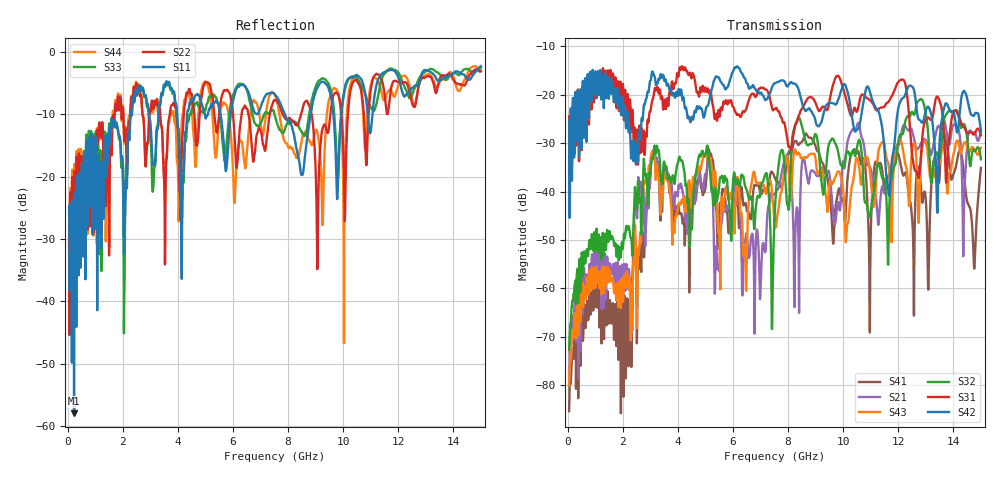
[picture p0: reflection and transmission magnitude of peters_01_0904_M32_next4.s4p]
# MHZ S RI R 50.00
! FREQ  S11  S12  S13  S14
!  S21  S22  S23  S24
!  S31  S32  S33  S34
!  S41  S42  S43  S44
!  REAL  IMAG  REAL  IMAG  REAL  IMAG  REAL  IMAG
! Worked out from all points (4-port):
!   1496 points, 50 MHz to 15 GHz, reference 50 ohm
!   strongest paths, dB at 50 MHz, 3.79 GHz, 7.53 GHz, 11.27 GHz, 15 GHz:
!     S42: -25.4, -20.0, -17.6, -23.3, -27.6
!     S31: -24.5, -17.2, -23.0, -23.1, -28.4
!     S32: -72.7, -37.2, -42.8, -34.2, -33.3
!     S43: -80.0, -49.1, -47.2, -32.1, -31.0
!     S21: -79.8, -40.5, -40.4, -46.8, -27.5
!     S41: -85.3, -43.2, -37.3, -34.4, -35.1
!   lowest |S11| = -57.9 dB at 230 MHz (marker M1), VSWR 1.00, Z = 50.1 + j0.0967 ohm
!   |S11| at or under -10 dB: start of sweep to 2.278 GHz; 3.967 GHz to 4.334 GHz (367 MHz wide, 8.84 % of centre); 7.879 GHz to 8.821 GHz (942.2 MHz wide, 11.3 % of centre)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
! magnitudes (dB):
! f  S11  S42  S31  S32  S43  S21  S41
! 50 MHz  -24.7  -25.4  -24.5  -72.7  -80.0  -79.8  -85.3
! 230 MHz  -57.9  -33.0  -29.8  -61.2  -67.7  -67.0  -73.2
! 2.26 GHz  -11.8  -27.2  -20.9  -48.8  -60.7  -60.3  -62.5
! 3.09 GHz  -17.9  -15.3  -20.9  -33.0  -32.1  -32.3  -31.9
! 7 GHz  -8.9  -19.6  -18.6  -40.1  -38.1  -60.0  -40.4
! 7.93 GHz  -10.5  -18.0  -27.7  -40.2  -32.8  -32.8  -34.7
! 15 GHz  -2.3  -27.6  -28.4  -33.3  -31.0  -27.5  -35.1
